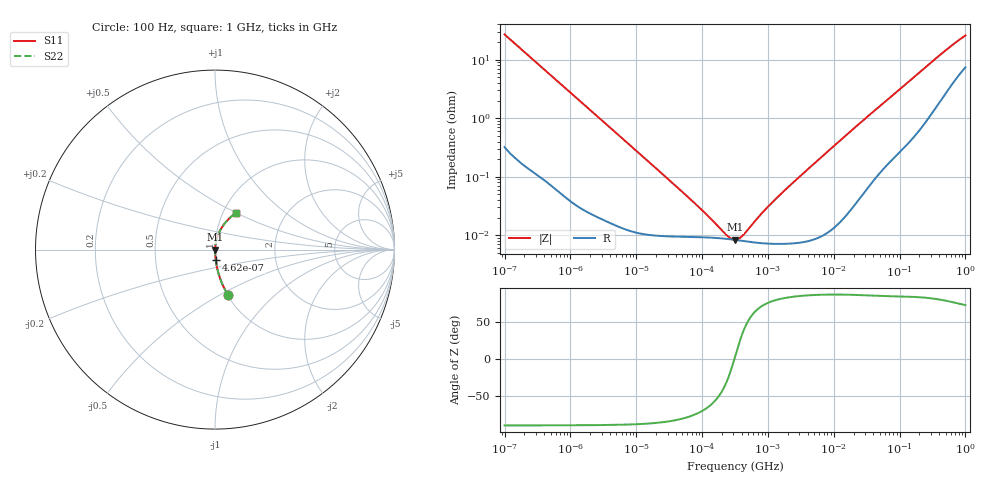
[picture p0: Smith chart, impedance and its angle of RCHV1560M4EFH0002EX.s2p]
! RCHV1560M4EFH0002EX  S-PARAMETER MODEL  (AEC-Q200 qualified)
! Model Generated by ELNA Corporation (http://www.ty-top.com)
! Version 1.0
! ELNA Control No. 240229
! Copyright (c) 2024 ELNA CO.,LTD. All Rights Reserved.
! Products Name : CONDUCTIVE POLYMER HYBRID ALUMINUM ELECTROLYTIC CAPACITORS
! Characteristics :
!  Capacitance  :  56uF  ,  Rated voltage  :  63V
!  Operating Temp. Range  :  -55 to +105 degC  ,  Endurance  :  10000hr at 105 degC
!  Dimension D  :  10mm  ,  Dimension L  :  10mm
! Frequency Range : 100Hz - 1GHz
! External Node Assignments :
!  1  o---| |---o  2
# MHz S RI R 50
!Freq[MHz].  S11 Real  S11 Imag  S21 Real  S21 Imag  S12 Real  S12 Imag  S22 Real  S22 Imag
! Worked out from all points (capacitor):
!   401 points, 100 Hz to 1 GHz, reference 50 ohm
!   read as one part in series: C = 58.9 uF near 108 Hz
!   lowest |Z| = 8.35 mohm at 316.2 kHz (marker M1)
!   series resonance near 308.3 kHz, so ESL is about 4.5 nH
!   S11 on the Smith chart (normalised r, x): 100 Hz: 1.01, -0.54; 462 Hz: 1.00, -0.12; 1 GHz: 1.15, +0.50
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0.0001  0.0706 -0.2503  0.9294 0.2503  0.9294 0.2503  0.0706 -0.2503
0.000113  0.0565 -0.2253  0.9435 0.2253  0.9435 0.2253  0.0565 -0.2253
0.000198  0.0197 -0.1335  0.9803 0.1335  0.9803 0.1335  0.0197 -0.1335
0.000462  0.00422 -0.0586  0.9958 0.0586  0.9958 0.0586  0.00422 -0.0586
0.001488  0.000621 -0.0184  0.9994 0.0184  0.9994 0.0184  0.000621 -0.0184
0.022131  9.91e-05 -0.00125  0.9999 0.00125  0.9999 0.00125  9.91e-05 -0.00125
0.090678  9.27e-05 -0.000283  0.9999 0.000283  0.9999 0.000283  9.27e-05 -0.000283
0.220039  8.74e-05 -6.43e-05  0.9999 6.43e-05  0.9999 6.43e-05  8.74e-05 -6.43e-05
0.248313  8.61e-05 -4.1e-05  0.9999 4.1e-05  0.9999 4.1e-05  8.61e-05 -4.1e-05
0.316228  8.33e-05 4.91e-06  0.9999 -4.91e-06  0.9999 -4.91e-06  8.33e-05 4.91e-06
0.386812  8.08e-05 4.44e-05  0.9999 -4.44e-05  0.9999 -4.44e-05  8.08e-05 4.44e-05
0.436516  7.92e-05 6.93e-05  0.9999 -6.93e-05  0.9999 -6.93e-05  7.92e-05 6.93e-05
0.767361  7.35e-05 0.00021  0.9999 -0.00021  0.9999 -0.00021  7.35e-05 0.00021
1.148154  7.15e-05 0.000352  0.9999 -0.000352  0.9999 -0.000352  7.15e-05 0.000352
2.018366  7.2e-05 0.000656  0.9999 -0.000656  0.9999 -0.000656  7.2e-05 0.000656
4.704354  8.51e-05 0.00156  0.9999 -0.00156  0.9999 -0.00156  8.51e-05 0.00156
21.75204  0.000402 0.00718  0.9996 -0.00718  0.9996 -0.00718  0.000402 0.00718
69.9842  0.00222 0.022  0.9978 -0.022  0.9978 -0.022  0.00222 0.022
184.0772  0.00853 0.0548  0.9915 -0.0548  0.9915 -0.0548  0.00853 0.0548
429.0422  0.0343 0.1171  0.9657 -0.1171  0.9657 -0.1171  0.0343 0.1171
695.825  0.0728 0.1671  0.9272 -0.1671  0.9272 -0.1671  0.0728 0.1671
1000  0.1163 0.2046  0.8837 -0.2046  0.8837 -0.2046  0.1163 0.2046
